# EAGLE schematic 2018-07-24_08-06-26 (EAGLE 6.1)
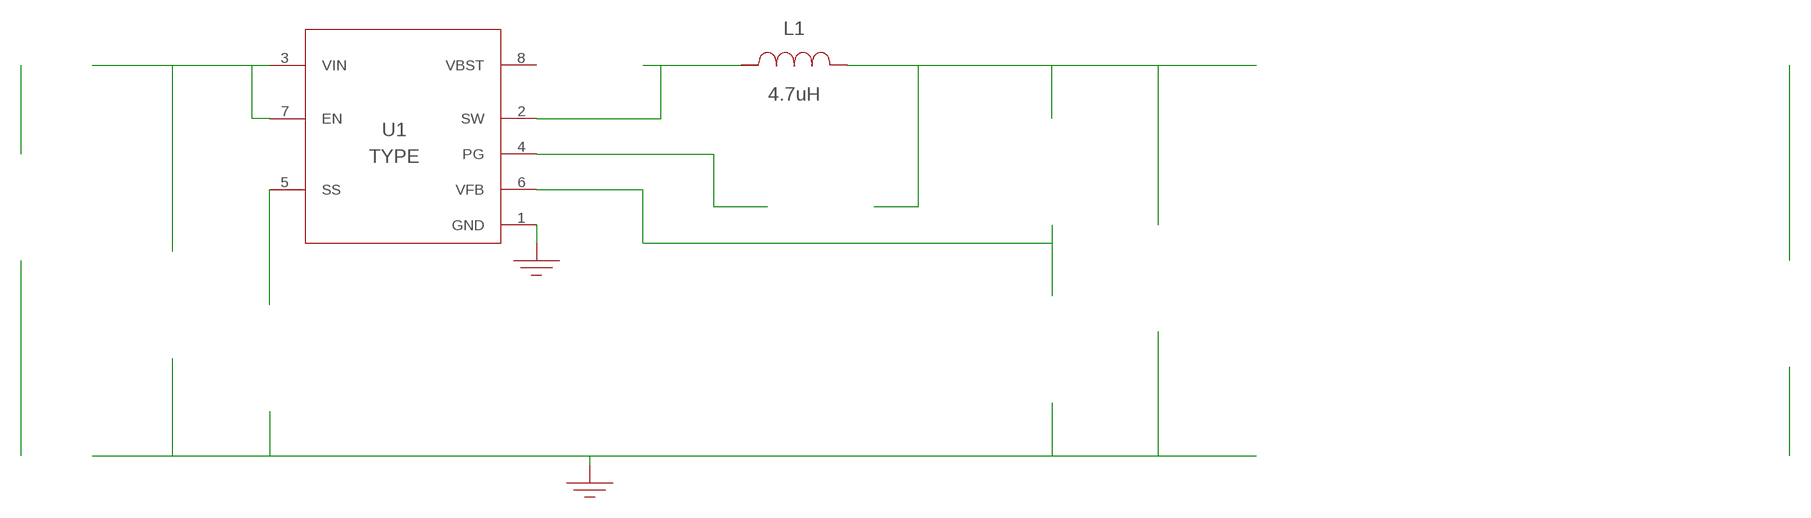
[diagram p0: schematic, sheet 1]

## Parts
CBST  100nF  C0603C104Z3VACTUC0603C104Z3VACTU  [0603]  (not placed on a sheet)
CIN  22uF  UUD1H220MCL1GSUUD1H220MCL1GS  [SM_RADIAL_6.3AMM]  (not placed on a sheet)
COUT  22uF  C1608X5R1A226M080ACC1608X5R1A226M080AC  [0603]  (not placed on a sheet)
CSS  8.2nF  GRM033R61A822KA01DGRM033R61A822KA01D  [0201]  (not placed on a sheet)
GND  WB_GND  WB_GNDWB_GND  [WB_GND]
GND2  WB_GND  WB_GNDWB_GND  [WB_GND]
IOUT  WB_CURRENT_LOAD  WB_CURRENT_LOADWB_CURRENT_LOAD  [WB_CURRENT_LOAD]  (not placed on a sheet)
L1  4.7uH  SRN6045-4R7YSRN6045-4R7Y  [SRN6045]
RFBB  10k  RMCF0402FT10K0RMCF0402FT10K0  [0402]  (not placed on a sheet)
RFBT  56.2k  RC0201FR-0756K2LRC0201FR-0756K2L  [0201]  (not placed on a sheet)
RPG  100k  ERJ-6ENF1003VERJ-6ENF1003V  [0805]  (not placed on a sheet)
U1  TPS562219DDFR  TPS562219DDFRTPS562219DDFR  [DDF0008A]
VIN  WB_BATTERY  WB_BATTERYWB_BATTERY  [WB_BATTERY]  (not placed on a sheet)

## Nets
0: Cin.-@2 Cout.2@2 Css.2@2 GND2.1 GND.1 Rfbb.2@2 U1.1(GND)
1: Cin.+@1 U1.3(VIN) U1.7(EN)
2: Rfbb.1@1 Rfbt.2@2 U1.6(VFB)
3: Rpg.2@2 U1.4(PG)
4: Cbst.1@1 L1.2 U1.2(SW)
5: Cout.1@1 L1.1 Rfbt.1@1 Rpg.1@1
6: Css.1@1 U1.5(SS)
7: Iout.+@1
8: Iout.-@2
9: Vin.+@1
10: Vin.-@2
11: Cbst.2@2 U1.8(VBST)
Unconnected: CBST.1 CBST.2 CIN.1(+) CIN.2(-) COUT.1 COUT.2 CSS.1 CSS.2 IOUT.1(+) IOUT.2(-) RFBB.1 RFBB.2 RFBT.1 RFBT.2 RPG.1 RPG.2 VIN.1(+) VIN.2(-)

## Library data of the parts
CBST = AcceleratedDesigns_Lib:C0603C104Z3VACTU; Cap: 1.0E-7; ESR: 0.0; IRMS: 0.0; Manufacturer_Name: Kemet; Manufacturer_Part_Number: C0603C104Z3VACTU; VDC: 25.0; Vendor: Kemet
CIN = AcceleratedDesigns_Lib:UUD1H220MCL1GS; Cap: 2.2E-5; ESR: 0.88; IRMS: 0.165; Manufacturer_Name: Nichicon; Manufacturer_Part_Number: UUD1H220MCL1GS; VDC: 50.0; Vendor: Nichicon
COUT = AcceleratedDesigns_Lib:C1608X5R1A226M080AC; Cap: 2.2E-5; Datasheet_URL: https://product.tdk.com/en/search/capacitor/ceramic/mlcc/info?part%5Fno%3DC1608X5R1A226M080AC; ESR: 0.00371; IRMS: 2.69936; Manufacturer_Name: TDK; Manufacturer_Part_Number: C1608X5R1A226M080AC; VDC: 10.0; Vendor: TDK
CSS = AcceleratedDesigns_Lib:GRM033R61A822KA01D; Cap: 8.2E-9; ESR: 0.0; IRMS: 0.0; Manufacturer_Name: MuRata; Manufacturer_Part_Number: GRM033R61A822KA01D; VDC: 10.0; Vendor: MuRata
GND GND2 = AcceleratedDesigns_Lib:WB_GND; Manufacturer_Name: WB_GND; Manufacturer_Part_Number: WB_GND; PowerPortType: POWER_GROUND; Value: Value
IOUT = AcceleratedDesigns_Lib:WB_CURRENT_LOAD; Manufacturer_Name: WB_CURRENT_LOAD; Manufacturer_Part_Number: WB_CURRENT_LOAD; PowerPortType: POWER_GROUND; Value: Value
L1 = AcceleratedDesigns_Lib:SRN6045-4R7Y; DCR: 0.0376; Datasheet_URL: http://www.bourns.com/data/global/pdfs/SRN6045.pdf; IDC: 3.0; L: 4.7E-6; Manufacturer_Name: Bourns; Manufacturer_Part_Number: SRN6045-4R7Y; Vendor: Bourns
RFBB = AcceleratedDesigns_Lib:RMCF0402FT10K0; Datasheet_URL: https://www.seielect.com/Catalog/SEI%2DRMCF%5FRMCP.pdf; Manufacturer_Name: Stackpole Electronics Inc; Manufacturer_Part_Number: RMCF0402FT10K0; Power: 0.063; Resistance: 10000.0; Tolerance: 1.0; Vendor: Stackpole Electronics Inc
RFBT = AcceleratedDesigns_Lib:RC0201FR-0756K2L; Datasheet_URL: http://www.yageo.com/documents/recent/PYu%2DRC%5FGroup%5F51%5FRoHS%5FL%5F5.pdf; Manufacturer_Name: Yageo; Manufacturer_Part_Number: RC0201FR-0756K2L; Power: 0.05; Resistance: 56200.0; Tolerance: 1.0; Vendor: Yageo America
RPG = AcceleratedDesigns_Lib:ERJ-6ENF1003V; Manufacturer_Name: Panasonic; Manufacturer_Part_Number: ERJ-6ENF1003V; Power: 0.125; Resistance: 100000.0; Tolerance: 1.0; Vendor: Panasonic
U1 = AcceleratedDesigns_Lib:TPS562219DDFR; CompType: IC; Manufacturer: Texas Instruments; Manufacturer_Name: Texas Instruments; Manufacturer_Part_Number: TPS562219DDFR; MountType: SMT; PIN_COUNT: 8; PackageReference: DDF0008A; PartNumber: TPS562219DDF; RefDes: RefDes; RoHS: Y; TYPE: TYPE; Value: Value
VIN = AcceleratedDesigns_Lib:WB_BATTERY; Manufacturer_Name: WB_BATTERY; Manufacturer_Part_Number: WB_BATTERY; PowerPortType: POWER_GROUND; Value: Value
